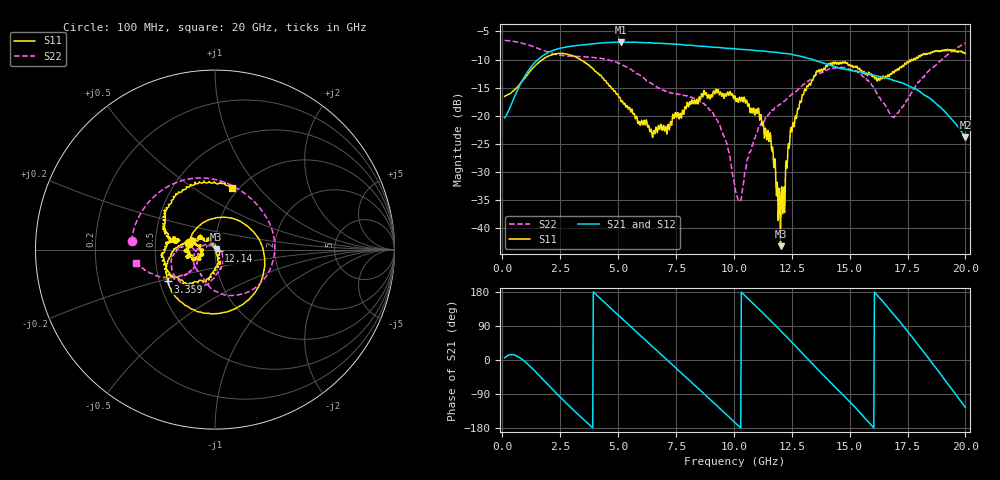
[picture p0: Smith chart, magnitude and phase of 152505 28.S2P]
!  2-Port S-parameters saved by WinCal
! VAR MeasName=S-Parameters (CALIBRATED_DATA) read from VNA (N5230C)
! VAR MeasDate=4/10/2015 9:31:07 AM
! VAR NAME=152505 28
! VAR FILENAME=152505 28.S2P
! VAR DATE=4/10/2015 9:31:07 AM
! VAR PHYS_PORTS=1,2
# Hz S DB R 50
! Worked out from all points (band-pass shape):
!   801 points, 100 MHz to 20 GHz, reference 50 ohm
!   highest |S21| = -6.88 dB at 5.125 GHz (marker M1); lowest = -23.8 dB at 20 GHz (marker M2)
!   |S21| within 3 dB of the highest: 1.573 GHz to 13.3 GHz (11.73 GHz wide, 158 % of centre)
!   lowest |S11| = -43.3 dB at 12.02 GHz (marker M3), VSWR 1.01, Z = 50.6 + j0.408 ohm
!   |S11| at or under -10 dB: start of sweep to 1.73 GHz; 3.373 GHz to 17.68 GHz (14.31 GHz wide, 136 % of centre); 17.70108 GHz to 17.76166 GHz (60.58 MHz wide, 0.342 % of centre)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
!   |S22| runs from -35.3 to -6.6 dB; largest |S21 - S12| = 0.0065
!   S11 on the Smith chart (normalised r, x): 100 MHz: 0.75, +0.06; 3.359 GHz: 0.55, -0.22; 12.14 GHz: 1.04, -0.02; 20 GHz: 0.93, +0.74
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1e8  -16.56 165.4  -20.37 5.8  -20.35 5.7  -6.61 174.2
8.21375e8  -14.00 61.3  -14.07 3.2  -14.06 3.1  -7.03 132.7
1.517875e9  -10.71 -18.2  -10.08 -36.1  -10.08 -36.1  -7.98 95.8
2.33875e9  -8.96 -86.8  -8.17 -88.2  -8.15 -88.2  -9.10 58.7
3.358625e9  -9.93 -146.1  -7.45 -148.4  -7.46 -148.4  -9.47 16.4
3.43325e9  -10.12 -150.0  -7.41 -152.6  -7.41 -152.6  -9.49 13.1
5.12475e9  -17.47 165.4  -6.88 111.7  -6.95 111.6  -10.88 -60.9
6.741625e9  -21.74 -173.5  -7.09 21.2  -7.09 21.0  -15.11 -110.7
8.532625e9  -16.94 -162.6  -7.62 -78.9  -7.59 -78.9  -17.46 -152.8
9.50275e9  -16.30 176.1  -7.92 -134.0  -7.90 -133.8  -22.77 162.7
1.005e10  -16.46 167.6  -8.09 -165.4  -8.10 -165.7  -32.76 102.8
1.027388e10  -17.09 160.4  -8.17 -178.1  -8.19 -178.2  -35.19 38.8
1.087088e10  -18.77 145.4  -8.36 146.8  -8.35 146.9  -24.14 -42.4
1.156738e10  -23.06 113.8  -8.64 105.1  -8.61 105.2  -19.32 -70.9
1.201512e10  -43.25 35.9  -8.84 77.6  -8.81 77.6  -17.97 -81.6
1.21395e10  -33.25 -26.2  -8.90 70.1  -8.90 70.0  -17.52 -85.0
1.25375e10  -21.63 -74.8  -9.12 44.8  -9.17 44.8  -16.13 -90.5
1.338325e10  -13.67 -117.3  -10.00 -9.2  -9.95 -8.9  -13.26 -109.3
1.477625e10  -10.45 -175.0  -11.72 -95.9  -11.70 -96.5  -11.44 -153.4
1.669162e10  -12.99 170.8  -13.39 135.7  -13.42 134.7  -19.33 -176.5
1.815925e10  -9.16 142.1  -16.14 23.8  -16.15 24.6  -13.13 -139.9
2e10  -8.91 74.7  -23.81 -125.3  -23.87 -124.3  -7.04 -170.3
